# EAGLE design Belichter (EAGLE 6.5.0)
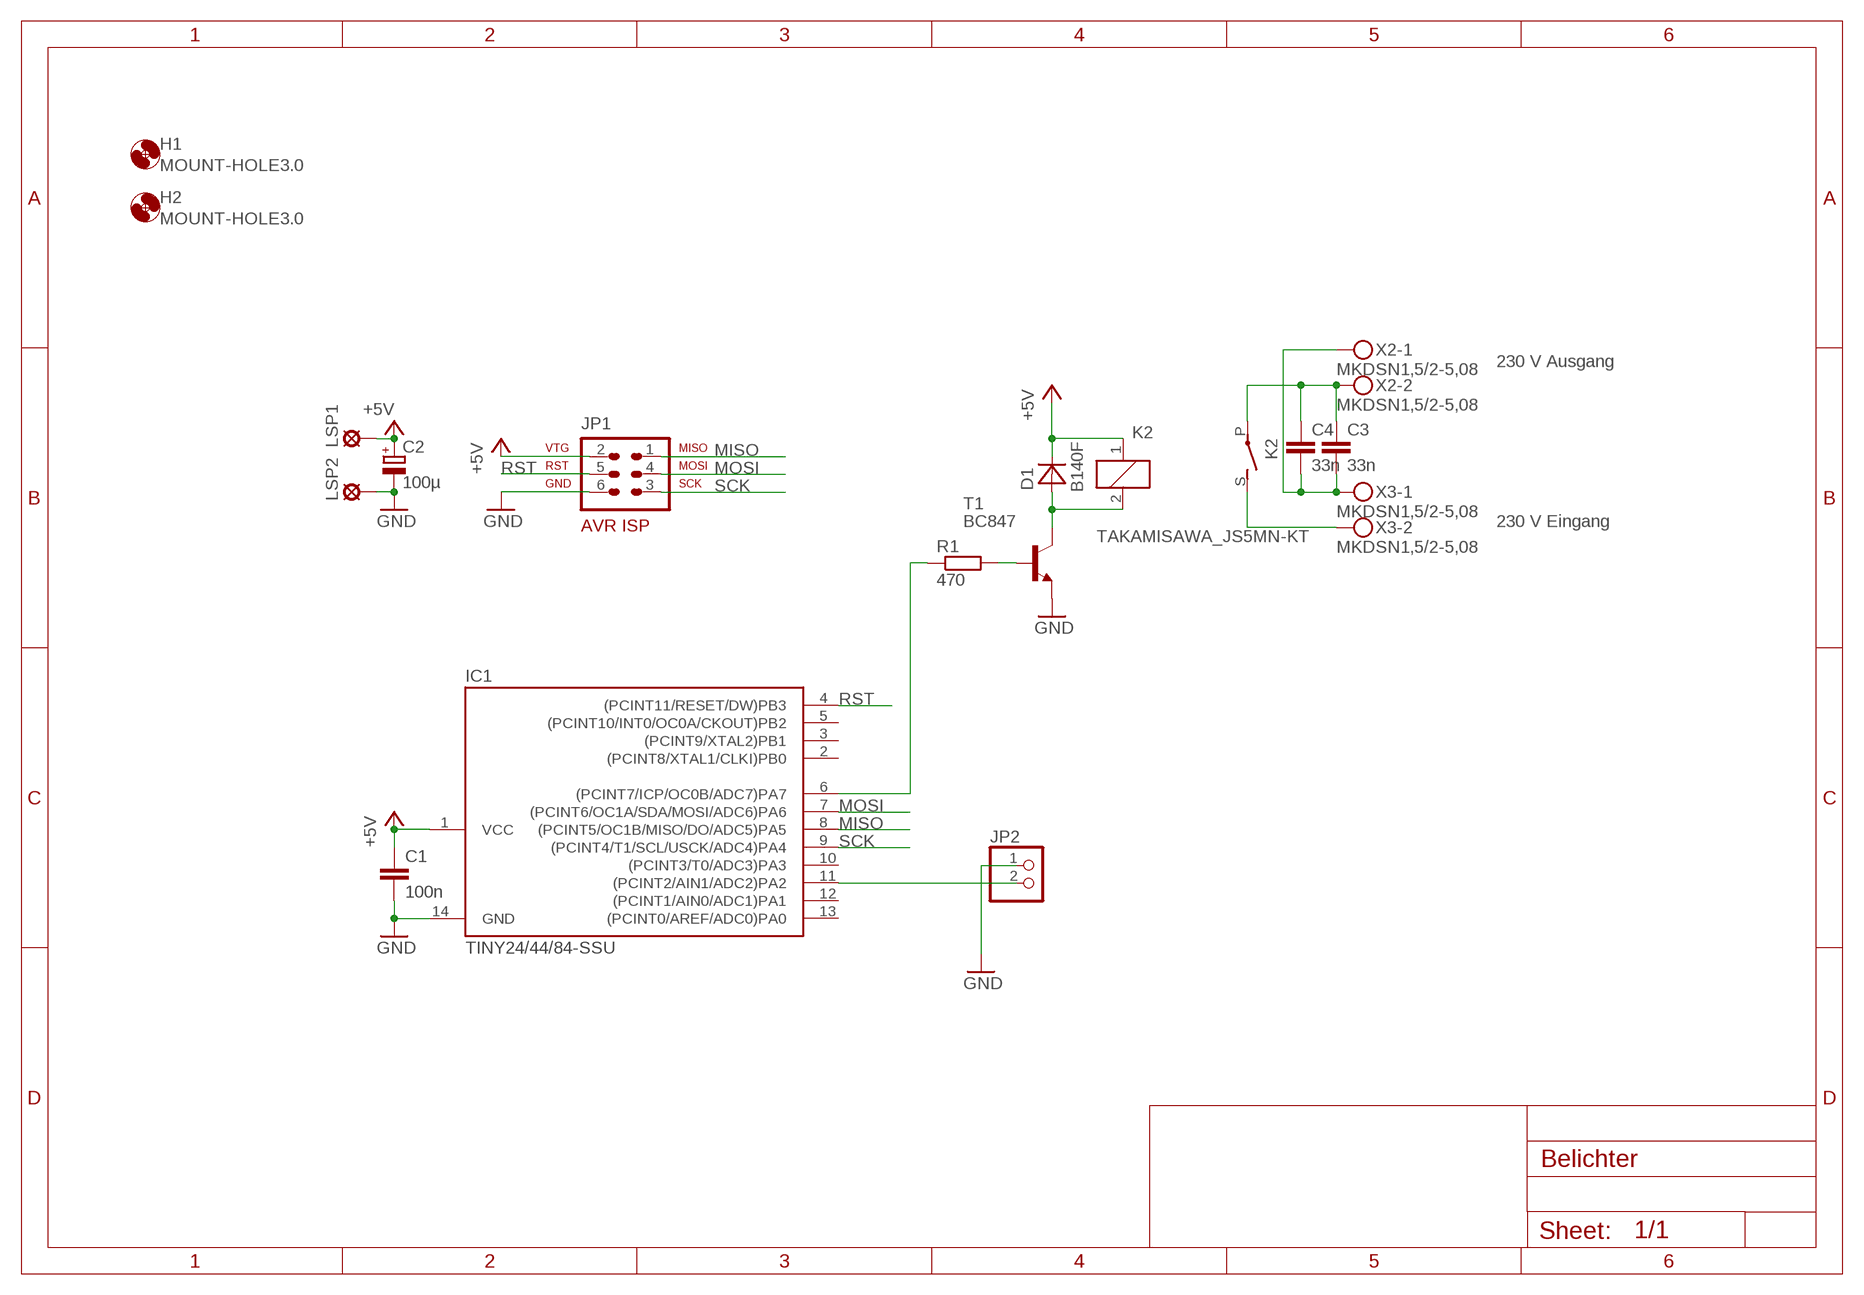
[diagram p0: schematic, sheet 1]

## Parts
C1  100n  C-EUC0805  [C0805]
C2  100µ  CPOL-EUE2-5  [E2-5]
C3  33n  C-EU102-043X133  [C102-043X133]
C4  33n  C-EU102-043X133  [C102-043X133]
D1  B140F  MBRA340T3  [SMA]
H1  MOUNT-HOLE3.0  [3,0]
H2  MOUNT-HOLE3.0  [3,0]
IC1  TINY24/44/84-SSU  [SOIC14]
JP1  AVR-ISP-6  [AVR-ISP-6]
JP2  PINHD-1X2  [1X02]
K2  TAKAMISAWA_JS5MN-KT  [TAKAMISAWA_JS5MN-KT]
LSP1  LSP10  [LSP10]
LSP2  LSP10  [LSP10]
R1  470  R-EU_R0805  [R0805]
T1  BC847  [SOT23]
X2  MKDSN1,5/2-5,08  [MKDSN1,5/2-5,08]
X3  MKDSN1,5/2-5,08  [MKDSN1,5/2-5,08]

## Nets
+5V: C1.1 C2.+ D1.C IC1.1(VCC) JP1.2 K2.1 LSP1.MP
GND: C1.2 C2.- IC1.14(GND) JP1.6 JP2.1 LSP2.MP T1.2(E)
MISO: IC1.8((PCINT5/OC1B/MISO/DO/ADC5)PA5) JP1.1
MOSI: IC1.7((PCINT6/OC1A/SDA/MOSI/ADC6)PA6) JP1.4
N$1: R1.2 T1.1(B)
N$2: D1.A K2.2 T1.3(C)
N$3: IC1.6((PCINT7/ICP/OC0B/ADC7)PA7) R1.1
N$4 [AC]: C3.2 C4.2 X2.1 X3.1
N$5 [AC]: K2.S(2:S) X3.2
N$7 [AC]: C3.1 C4.1 K2.P(2:P) X2.2
N$14: IC1.11((PCINT2/AIN1/ADC2)PA2) JP2.2
RST: IC1.4((PCINT11/RESET/DW)PB3) JP1.5
SCK: IC1.9((PCINT4/T1/SCL/USCK/ADC4)PA4) JP1.3
Unconnected: IC1.2((PCINT8/XTAL1/CLKI)PB0) IC1.3((PCINT9/XTAL2)PB1) IC1.5((PCINT10/INT0/OC0A/CKOUT)PB2) IC1.10((PCINT3/T0/ADC3)PA3) IC1.12((PCINT1/AIN0/ADC1)PA1) IC1.13((PCINT0/AREF/ADC0)PA0)

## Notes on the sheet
- 230 V Ausgang
- 230 V Eingang

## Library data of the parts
C1 C3 C4 = rcl:C-EU: CAPACITOR, European symbol
C2 = rcl:CPOL-EU: POLARIZED CAPACITOR, European symbol
D1 = diode:MBRA340T3: Surface Mount Schottky Power Rectifier
H1 H2 = holes:MOUNT-HOLE: MOUNTING HOLE with drill center marker
IC1 = avr-4:TINY24/44/84
JP1 = avr-4:AVR-ISP-6: AVR ISP-6 Serial Programming Header
JP2 = pinhead:PINHD-1X2: PIN HEADER
K2 = eigene:TAKAMISAWA_JS5MN-KT: RELAY 1 x norm. open, Omron
LSP1 LSP2 = solpad:LSP10: SOLDER PAD
R1 = rcl:R-EU_: RESISTOR, European symbol
T1 = transistor:BC847: NPN TRANSISTOR
X2 X3 = con-phoenix-508:MKDSN1,5/2-5,08: MKDSN 1,5/ 2-5,08 Printklemme; MPN: MKDSN 1,5/2-5.08; OC_FARNELL: 1792903; OC_NEWARK: 30M2397

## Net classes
1 AC: clearance 5 mm to class 0, clearance 0.6 mm

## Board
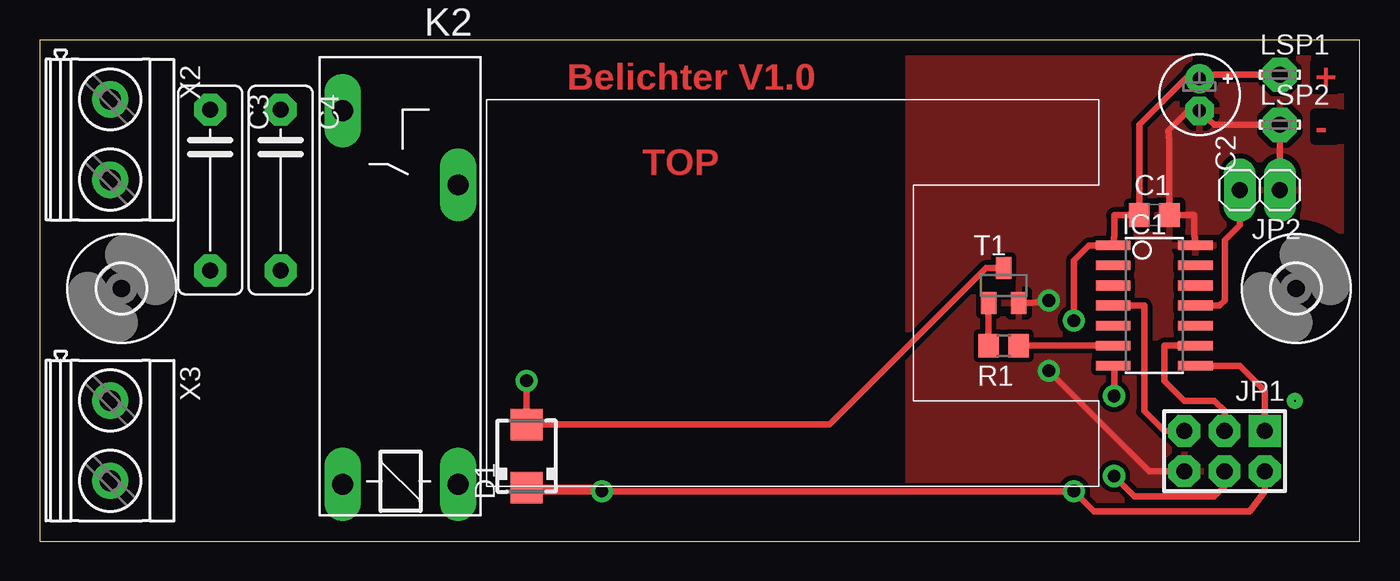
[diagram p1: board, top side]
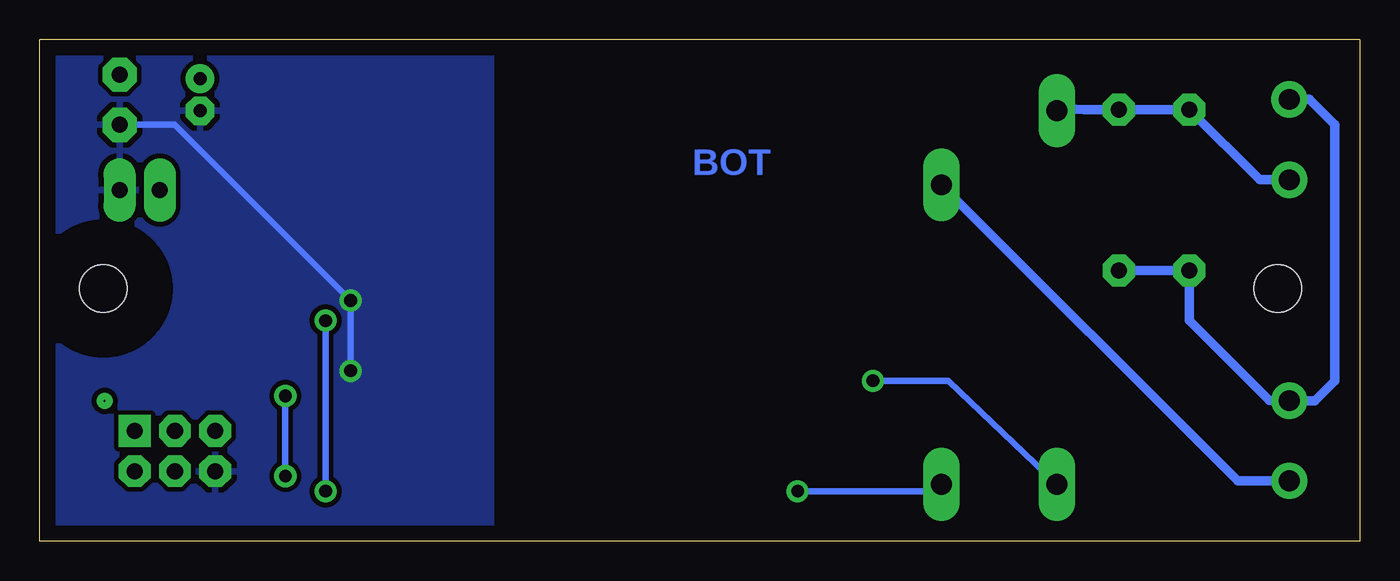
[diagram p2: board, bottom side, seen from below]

Size 83.49 x 31.75 mm. Coordinates in mm from the lower left corner, seen from the top.
Outline: 83.49,31.74 83.49,0 0,0 0,31.74
Outline: 0,31.75 83.49,31.75
Copper layers (1*16): Top 0.035mm / dielectric 1.5mm / Bottom 0.035mm
Design rules: minimum track width 0.3mm, minimum drill 0.8mm, track to track 0.2mm, track to pad 0.2mm, pad to pad 0.2mm, via to via 0.2mm, smd to smd 0.2mm, copper to edge 1mm, drill to drill 1mm, minimum pad ring 0.5mm, minimum via ring 0.3mm, stop-mask expansion 4mil, vias tented up to drill 0mil, thermal gap 14mil

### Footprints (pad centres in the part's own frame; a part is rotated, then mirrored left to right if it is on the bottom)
C0805 = smd 1.3 x 1.5: 1 -0.95,0; 2 0.95,0
E2-5 = drill 0.813 pad 1.27: + -1.016,0 | drill 0.813 pad 1.27 octagon: - 1.016,0
C102-043X133 = drill 1.016 octagon: 1 -5.08,0; 2 5.08,0
SMA = smd 2 x 2: A 2,0; C -2,0
3,0 = hole 3: 0,0
SOIC14 = smd 0.61 x 2.21: 1 -3.81,-2.603; 2 -2.54,-2.603; 3 -1.27,-2.603; 4 0,-2.603; 5 1.27,-2.603; 6 2.54,-2.603; 7 3.81,-2.603; 8 3.81,2.603; 9 2.54,2.603; 10 1.27,2.603; 11 0,2.603; 12 -1.27,2.603; 13 -2.54,2.603; 14 -3.81,2.603
AVR-ISP-6 = drill 1.016 square: 1 -2.54,-1.27 | drill 1.016 octagon: 2 -2.54,1.27; 3 0,-1.27; 4 0,1.27; 5 2.54,-1.27; 6 2.54,1.27
1X02 = drill 1.016 long: 1 -1.27,0; 2 1.27,0
TAKAMISAWA_JS5MN-KT = drill 1.321 long: 1 -4.01,-5.183; 2 -4.01,2.11; P 19.63,2.11; S 14.935,-5.183
LSP10 = drill 1.016 pad 2.159 octagon: MP 0,0
R0805 = smd 1.3 x 1.5: 1 -0.95,0; 2 0.95,0
SOT23 = smd 1 x 1.4: 1 -0.95,-1.1; 2 0.95,-1.1; 3 0,1.1
MKDSN1,5/2-5,08 = drill 1.3 pad 2: 1 -2.561,0.025; 2 2.519,0.025

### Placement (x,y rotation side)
C1  70.48,20.64 0 top
C2  73.34,28.26 270 top
C3  10.79,22.23 270 top
C4  15.24,22.23 270 top
D1  30.8,5.4 90 top
H1  79.45,16 0 top
H2  5.18,16 0 top
IC1  70.48,14.92 270 top
JP1  74.93,5.71 180 top
JP2  77.15,22.23 180 top
K2  21.27,7.62 90 top
LSP1  78.42,29.53 0 top
LSP2  78.42,26.35 0 top
R1  60.96,12.38 180 top
T1  60.96,16.19 0 top
X2  4.45,25.4 270 top
X3  4.45,6.35 270 top

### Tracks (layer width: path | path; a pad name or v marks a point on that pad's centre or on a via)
+5V  (via drill 0.8)
  Top 0.406: v65.41,13.97 65.41,17.78 66.36,18.73 IC1.1 67.94,19.43 67.94,20.64 C1.1 69.53,21.91 69.53,26.35 72.45,29.27 C2.+ 73.6,29.53 LSP1.MP | JP1.2 77.47,3.17 76.52,1.91 66.67,1.91 v65.41,3.17 v35.56,3.17 | v35.56,3.17 31.02,3.17 D1.C 35.34,3.4 v35.56,3.17
  Bottom 0.406: v65.41,3.17 v65.41,13.97 | v35.56,3.17 26.57,3.17 K2.1
GND  (via drill 0.8)
  Top 0.406: IC1.14 73.03,19.43 73.03,20.64 C1.2 71.44,22.23 71.44,25.4 71.37,25.97 72.64,27.24 C2.- 73.66,26.92 74.3,26.35 LSP2.MP JP2.1 | T1.2 62.72,15.09 v63.82,15.24 | JP1.6 70.17,4.45 v63.82,10.79
  Bottom 0.406: LSP2.MP 74.93,26.35 v63.82,15.24 v63.82,10.79
  pour Top (isolate 0.305): 83.5,0 83.5,32.07 54.93,32.07 54.93,0
  pour Bottom (isolate 0.305): 83.5,31.75 83.5,0 54.93,0 54.93,31.75
MISO
  Top 0.406: IC1.8 75.88,11.11 77.47,9.53 JP1.1
MOSI  (via drill 0.8)
  Top 0.406: JP1.4 74.93,3.49 74.3,2.86 69.22,2.86 v67.94,4.13 | v67.94,9.21 67.94,11.11 IC1.7
  Bottom 0.406: v67.94,4.13 v67.94,9.21
N$1
  Top 0.406: R1.2 T1.1
N$2  (via drill 0.8)
  Top 0.406: T1.3 59.84,17.29 49.94,7.4 D1.A v30.8,10.16
  Bottom 0.406: v30.8,10.16 26.03,10.16 K2.2
N$3
  Top 0.406: IC1.6 R1.1
N$4
  Bottom 0.61: C4.2 C3.2 10.79,13.97 5.74,8.91 X3.1 4.45,8.89 2.86,8.89 1.59,10.16 1.59,26.35 3.2,27.96 X2.1
N$5
  Bottom 0.61: X3.2 7.73,3.83 K2.S
N$6  (via drill 0.1 pad 1.02)
  other vias: 79.38,8.89
N$7
  Bottom 0.61: X2.2 6.33,22.88 C3.1 C4.1 17.46,27.3 18.94,27.42 19.16,27.42 K2.P
N$14
  Top 0.406: IC1.11 74.61,14.92 74.93,15.24 74.93,19.05 75.88,20 JP2.2
RST
  Top 0.406: IC1.4 69.85,14.92 69.85,8.26 71.12,6.99 JP1.5
SCK
  Top 0.406: IC1.9 71.12,12.38 71.12,10.16 72.39,8.89 74.3,8.89 74.93,8.26 JP1.3

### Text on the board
Top: Belichter V1.0 | + | - | TOP
Bottom: BOT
